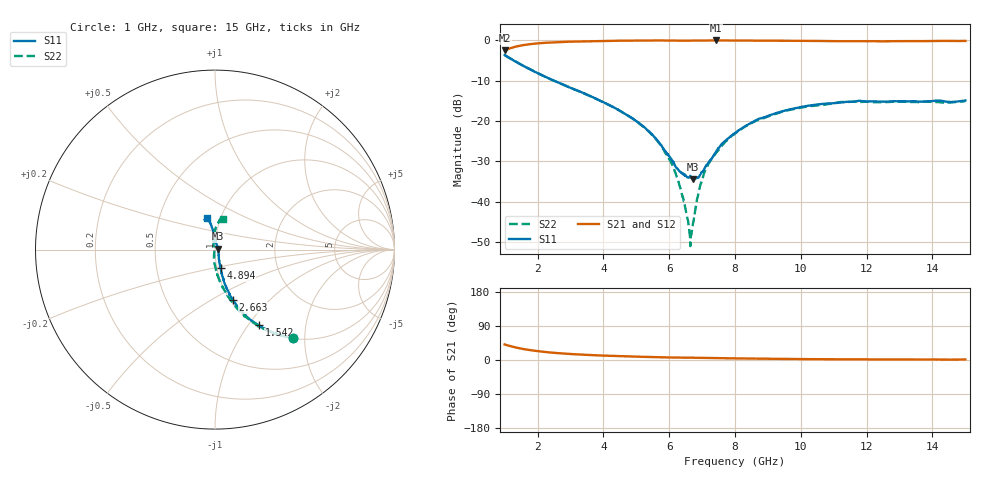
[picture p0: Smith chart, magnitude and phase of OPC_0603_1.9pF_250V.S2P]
! FILE NAME
! DATE 08/20/2012  13:55
! CORRECTED  DATA
# GHz  S  MA  R  50.00
!  FREQ  S11M  S11A  S21M  S21A  S12M  S12A  S22M  S22A
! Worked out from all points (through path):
!   1601 points, 1 GHz to 15 GHz, reference 50 ohm
!   highest |S21| = -0.05 dB at 7.423 GHz (marker M1); lowest = -2.5 dB at 1 GHz (marker M2)
!   group delay of S21, straight-line fit = 4.83 ps
!   lowest |S11| = -34.5 dB at 6.714 GHz (marker M3), VSWR 1.04, Z = 51.8 + j0.594 ohm
!   |S11| at or under -10 dB: 2.496 GHz to end of sweep
!   |S22| runs from -51.0 to -3.7 dB; largest |S21 - S12| = 0.0084
!   S11 on the Smith chart (normalised r, x): 1 GHz: 1.02, -1.75; 1.542 GHz: 1.02, -1.13; 2.663 GHz: 1.03, -0.63; 4.894 GHz: 1.04, -0.22; 15 GHz: 0.86, +0.31
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1  0.6558 -48.5  0.7488 41.1  0.7482 41.1  0.6557 -48.6
1.5425  0.4878 -60.0  0.867 29.4  0.8657 29.4  0.4877 -60.4
2.6625  0.2962 -70.5  0.9489 17.8  0.9475 17.8  0.295 -72.6
3.33625  0.2271 -73.2  0.9689 14.2  0.9679 14.2  0.2261 -77.5
4.89375  0.1071 -73.1  0.9897 9.1  0.989 9.1  0.1065 -88.0
5.6725  0.05521 -67.0  0.9935 7.3  0.9929 7.3  0.05431 -96.1
6.13625  0.0308 -47.0  0.9909 6.5  0.9898 6.2  0.02618 -102.3
6.4075  0.02228 -19.2  0.9879 6.2  0.9877 6.2  0.01145 -104.8
6.6175  0.02012 5.9  0.9882 6.0  0.9878 6.0  0.004094 -141.7
6.67  0.01974 9.9  0.9885 6.0  0.9879 6.0  0.003858 -162.1
6.71375  0.01892 17.6  0.9895 6.0  0.989 6.0  0.005037 164.6
6.87125  0.0198 38.0  0.9913 5.8  0.9908 5.8  0.01172 126.5
7.01125  0.02345 55.7  0.9921 5.6  0.9915 5.6  0.01913 113.3
7.16  0.02913 68.6  0.993 5.4  0.9919 5.4  0.02743 106.9
7.4225  0.04136 83.9  0.9944 5.0  0.9926 5.0  0.04002 101.2
8  0.07086 91.7  0.9927 4.3  0.9919 4.3  0.06973 96.4
8.72625  0.1064 95.5  0.9903 3.6  0.9896 3.6  0.1033 90.1
9.51375  0.1341 98.6  0.9861 2.9  0.9854 2.8  0.1325 86.5
10.33625  0.1565 100.5  0.9817 2.2  0.9807 2.2  0.153 82.3
11.255  0.1698 103.5  0.9727 1.8  0.9725 1.8  0.1721 79.5
12.6725  0.1739 107.2  0.97 1.6  0.9691 1.6  0.1716 76.4
15  0.1797 104.3  0.9812 1.5  0.9802 1.5  0.1769 75.2
